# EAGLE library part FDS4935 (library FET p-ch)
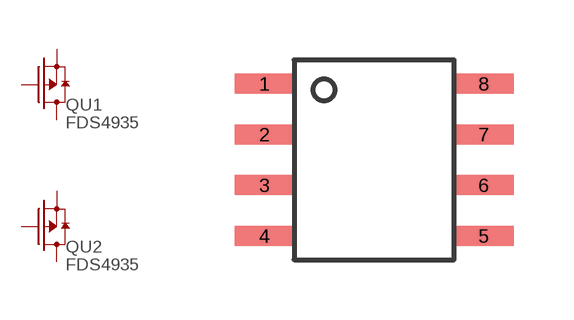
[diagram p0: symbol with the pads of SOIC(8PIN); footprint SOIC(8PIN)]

Designator prefix Q; gates U1=DUALDRAIN U2=DUALDRAIN

## FDS4935  [SOIC(8PIN)]
1  U1:S  pas
2  U1:G  pas
3  U2:S  pas
4  U2:G  pas
5  U2:D2  pas
6  U2:D1  pas
7  U1:D2  pas
8  U1:D1  pas

## Footprint SOIC(8PIN) (pad centres in mm)
4*5mm size , 0.05inch pitch , 8pin pacage
smd 1.5 x 0.5: 1 -2.74,1.905; 2 -2.74,0.635; 3 -2.74,-0.635; 4 -2.74,-1.905; 5 2.74,-1.905; 6 2.74,-0.635; 7 2.74,0.635; 8 2.74,1.905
